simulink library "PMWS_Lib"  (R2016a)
settings: Solver=ode45  StartTime=0.0  StopTime=10.0  RelTol=1e-3
libraries: nesl_utility x4, PMWS_Simscape_Library_lib x1

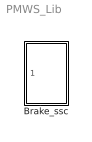
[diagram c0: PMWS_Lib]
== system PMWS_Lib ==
  Brake_ssc : Subsystem

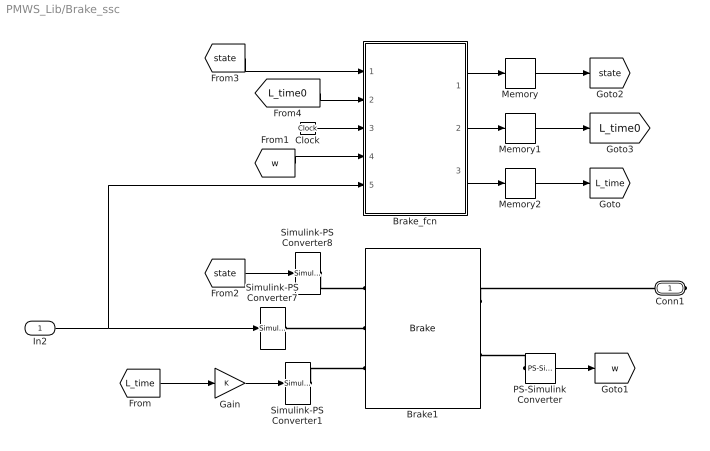
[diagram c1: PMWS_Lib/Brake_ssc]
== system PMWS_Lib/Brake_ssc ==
  In2 : Inport
  Brake1 : PMWS_Simscape_Library_lib/Chassis/Brake  w_thr=1.0 rad/s  Brake_force_thr=0.1 N  T_L=0.1 s  uk=1.0  Er=1.0 m  w_T_specify=off  w_T_priority=None  w_T=0 rad/s  t_F_specify=off  t_F_priority=None  t_F=0 N*m  t_T_specify=off  t_T_priority=None  t_T=0 N*m  state_specify=off  state_priority=None  state=0
  Brake_fcn : MATLAB Function  TreatAsAtomicUnit=on
  Clock : Clock
  Gain : Gain
  Memory : Memory  X0=1
  Memory1 : Memory  X0=1
  Memory2 : Memory  X0=1
  PS-Simulink Converter : nesl_utility/PS-Simulink Converter  PhysicalDomain=network_engine_domain  SubClassName=ps_output  LeftPortType=input  RightPortType=output  PseudoPeriodic=off  Frequencies=[]  Unit=1  AffineConversion=off
  Simulink-PS Converter1 : nesl_utility/Simulink-PS Converter  PhysicalDomain=network_engine_domain  SubClassName=ps_input  LeftPortType=input  RightPortType=output  PseudoPeriodic=off  Frequencies=[]  NoiseDistribution=none  NoiseParameters=[]  Unit=s  AffineConversion=off  InputFiltering=off  SimscapeFilterOrder=1  InputFilterTimeConstant=0.1  UdotUserProvided=1
  Simulink-PS Converter7 : nesl_utility/Simulink-PS Converter  PhysicalDomain=network_engine_domain  SubClassName=ps_input  LeftPortType=input  RightPortType=output  PseudoPeriodic=off  Frequencies=[]  NoiseDistribution=none  NoiseParameters=[]  Unit=N  AffineConversion=off  InputFiltering=off  SimscapeFilterOrder=1  InputFilterTimeConstant=0.1  UdotUserProvided=1
  Simulink-PS Converter8 : nesl_utility/Simulink-PS Converter  PhysicalDomain=network_engine_domain  SubClassName=ps_input  LeftPortType=input  RightPortType=output  PseudoPeriodic=off  Frequencies=[]  NoiseDistribution=none  NoiseParameters=[]  Unit=1  AffineConversion=off  InputFiltering=off  SimscapeFilterOrder=1  InputFilterTimeConstant=0.1  UdotUserProvided=1
  Conn1 : PMIOPort  Port=1  Side=Right
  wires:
  Memory/1 -> [state]
  In2/1 -> Brake_fcn/5(Brake), Simulink-PS Converter7/1
  Brake_fcn/1(state_out) -> Memory/1
  Clock/1 -> Brake_fcn/3(time)
  Brake_fcn/2(L_time0_out) -> Memory1/1
  Brake_fcn/3(L_time) -> Memory2/1
  [L_time] -> Gain/1
  Memory2/1 -> [L_time]
  Gain/1 -> Simulink-PS Converter1/1
  PS-Simulink Converter/1 -> [w]
  [w] -> Brake_fcn/4(w)
  [state] -> Simulink-PS Converter8/1
  [state] -> Brake_fcn/1(state_in)
  Memory1/1 -> [L_time0]
  [L_time0] -> Brake_fcn/2(L_time0_in)
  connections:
  Simulink-PS Converter8/RConn1 -- Brake1/LConn1
  Brake1/RConn1 -- Conn1/RConn1
  PS-Simulink Converter/LConn1 -- Brake1/RConn2
  Simulink-PS Converter7/RConn1 -- Brake1/LConn2
  Simulink-PS Converter1/RConn1 -- Brake1/LConn3

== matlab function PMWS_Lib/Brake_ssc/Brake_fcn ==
function [state_out,L_time0_out,L_time] = fcn(state_in,L_time0_in,time, w,Brake)

%#codegen

w_thr = 1.0;
Brake_thr = 0.1;


if(w>= 0)&& (w<= w_thr) && (Brake > Brake_thr)
 state_out=0;
elseif(w>= 0)&&(w <= w_thr) && (Brake < Brake_thr)
 state_out=1;
 
elseif(w >= w_thr)&& (Brake > Brake_thr)
 state_out=1;
elseif(w >= w_thr)&& (Brake < Brake_thr)
 state_out=2;

elseif(w < 0) && (w >= -w_thr)&& (Brake < Brake_thr)
 state_out=-1;
elseif(w < 0) && (w >= -w_thr)&& (Brake > Brake_thr)
 state_out=0;

else
 state_out=2;
end



if(state_in == 1)&&(state_out == 0) 
    L_time0_out=time;
    L_time = 0;
elseif(state_in == -1)&&(state_out == 0) 
    L_time0_out=time;
    L_time = 0;

elseif(state_in ==0)&&(state_out == 0)
     L_time0_out=L_time0_in;
    L_time = min(time- L_time0_out, 1);
    
else
    L_time0_out = 0;
    L_time = 0;
    
       
end
